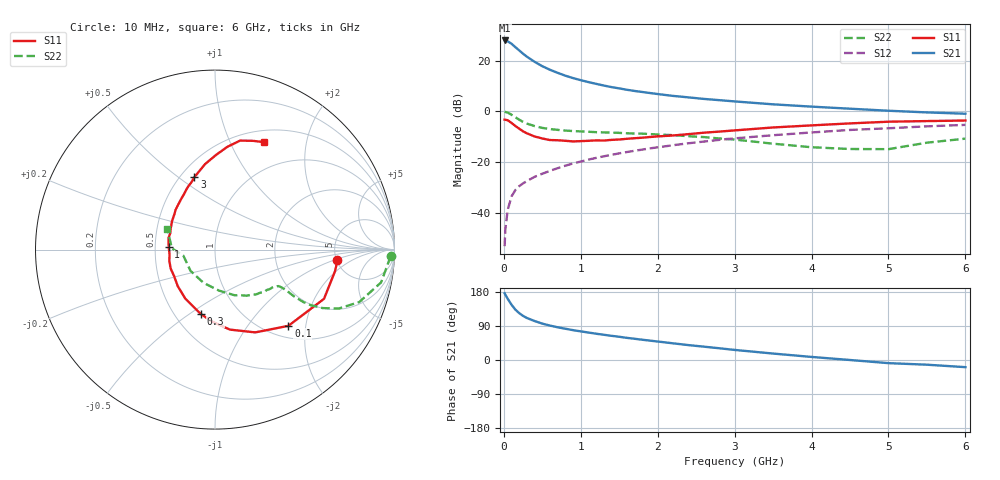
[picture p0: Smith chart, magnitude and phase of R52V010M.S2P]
! SIEMENS Small Signal Semiconductors
! BFR183
! Si NPN RF Bipolar Junction Transistor in SOT23
! VCE = 2 V  IC = 10 mA
! Common Emitter S-Parameters:  May  1996
# GHz  S  MA  R  50
!  f  S11  S21  S12  S22
! GHz  MAG  ANG  MAG  ANG  MAG  ANG  MAG  ANG
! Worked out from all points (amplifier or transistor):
!   36 points, 10 MHz to 6 GHz, reference 50 ohm
!   highest |S21| = 27.9 dB at 10 MHz (marker M1)
!   |S21| within 3 dB of that: start of sweep to 163.6 MHz
!   unconditionally stable (mu >= 1): 758.3 MHz to 2.504 GHz
!   at 250 MHz: K = 0.63, MSG = 25.5 dB, |S12| = -28.4 dB
!   at 1.4 GHz: K = 1.06, MAG = 11.9 dB, |S12| = -17.2 dB
!   at 6 GHz: K = 0.90, MSG = 2.2 dB, |S12| = -5.4 dB
!   lowest NFmin = 1.30 dB at 450 MHz
!   S11 on the Smith chart (normalised r, x): 10 MHz: 5.08, -1.14; 100 MHz: 1.23, -1.60; 300 MHz: 0.67, -0.56; 1 GHz: 0.59, +0.02; 3 GHz: 0.59, +0.58; 6 GHz: 0.64, +1.34
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0.01  0.6851 -5.0  24.85 176.2  0.0022 89.0  0.9789 -2.2
0.02  0.6795 -10.2  24.53 172.2  0.0048 82.5  0.9671 -4.6
0.05  0.6665 -24.3  23.87 161.6  0.0114 79.5  0.9431 -11.2
0.1  0.5895 -46.1  21.41 145.8  0.021 70.8  0.8551 -20.0
0.15  0.5127 -64.1  18.31 132.9  0.0281 65.8  0.763 -25.5
0.2  0.4536 -79.4  15.81 123.6  0.0335 63.2  0.683 -28.5
0.25  0.4025 -92.0  13.62 116.4  0.038 62.0  0.6184 -30.1
0.3  0.3677 -102.4  11.88 110.8  0.0422 61.9  0.572 -30.7
0.4  0.3189 -121.3  9.437 102.8  0.0511 62.2  0.5112 -30.6
0.5  0.2911 -135.4  7.728 96.0  0.0588 63.5  0.4706 -30.0
0.6  0.2713 -147.3  6.571 90.8  0.0671 64.2  0.4462 -29.7
0.7  0.2686 -156.8  5.714 86.3  0.0757 65.1  0.4303 -29.6
0.8  0.2621 -166.3  5.026 82.5  0.0847 64.9  0.4169 -29.7
1  0.258 177.1  4.098 75.5  0.1022 65.1  0.4013 -30.6
1.1  0.262 171.0  3.758 72.5  0.1116 64.9  0.3947 -31.6
1.6  0.2871 146.5  2.651 58.4  0.1574 62.5  0.3684 -37.3
2.2  0.3338 125.6  2.008 44.0  0.2145 57.5  0.3389 -47.4
3  0.42 105.8  1.564 26.6  0.2925 48.7  0.2771 -66.7
3.5  0.4799 96.6  1.371 17.0  0.3376 42.4  0.2299 -84.3
4.5  0.5772 83.1  1.124 0.0  0.4289 29.8  0.1806 -139.1
5.5  0.641 71.0  0.95 -12.4  0.5048 17.8  0.2408 178.2
6  0.6574 65.7  0.895 -18.9  0.5397 10.0  0.2889 156.5
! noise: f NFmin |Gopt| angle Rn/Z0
0.45  1.3  0.15  45  0.18
0.9  1.4  0.2  125  0.19
1.8  2.1  0.34  -170  0.14
